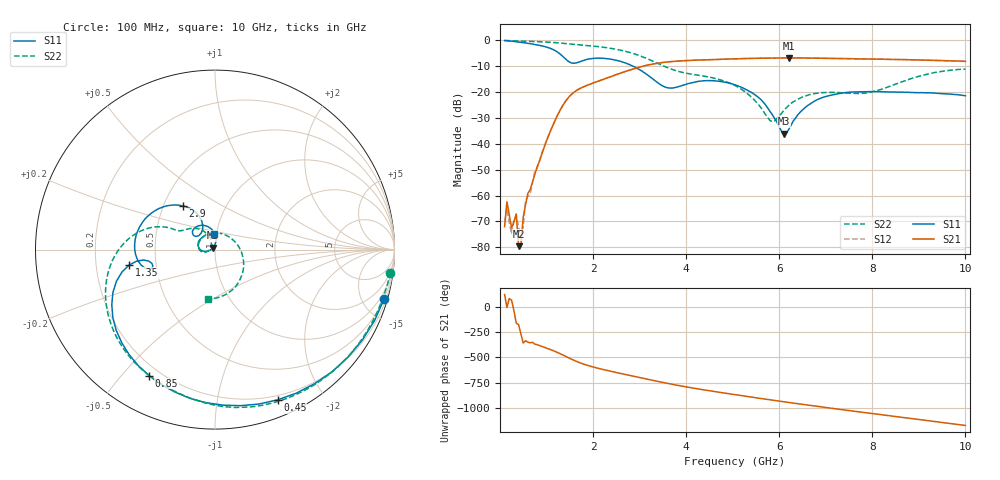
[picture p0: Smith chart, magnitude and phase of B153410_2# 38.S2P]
!  2-Port S-parameters saved by WinCal
! VAR MeasName=S-Parameters (CALIBRATED_DATA) read from VNA (N5245A)
! VAR MeasDate=2016-12-23 10:01:18
! VAR NAME=B153410_2# 38
! VAR FILENAME=B153410_2# 38.S2P
! VAR DATE=2016-12-23 10:01:18
! VAR PHYS_PORTS=1,2
# Hz S DB R 50
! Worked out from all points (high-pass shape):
!   199 points, 100 MHz to 10 GHz, reference 50 ohm
!   highest |S21| = -6.85 dB at 6.2 GHz (marker M1); lowest = -79.6 dB at 400 MHz (marker M2)
!   |S21| within 3 dB of the highest: 3.122 GHz to end of sweep
!   lowest |S11| = -36.1 dB at 6.1 GHz (marker M3), VSWR 1.03, Z = 49 + j1.14 ohm
!   |S11| at or under -10 dB: 2.852 GHz to end of sweep
!   |S22| runs from -31.5 to -0.1 dB; largest |S21 - S12| = 0.0033
!   S11 on the Smith chart (normalised r, x): 100 MHz: 0.46, -7.01; 450 MHz: 0.16, -1.49; 850 MHz: 0.16, -0.59; 1.35 GHz: 0.35, -0.08; 2.9 GHz: 0.63, +0.34; 10 GHz: 0.98, +0.17
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1e8  -0.16 -16.2  -72.01 124.3  -70.36 178.4  -0.13 -7.4
1.5e8  -0.24 -23.9  -62.42 -4.4  -64.98 -8.7  -0.17 -10.9
2.5e8  -0.42 -39.0  -72.53 68.3  -74.87 -42.4  -0.25 -17.7
3.5e8  -0.62 -53.5  -67.12 -160.2  -67.50 -9.8  -0.31 -24.3
4e8  -0.73 -60.5  -79.56 -174.6  -72.11 51.5  -0.33 -27.6
4.5e8  -0.85 -67.4  -79.07 93.5  -76.23 14.4  -0.36 -30.9
5e8  -0.97 -74.1  -68.38 2.5  -72.33 102.4  -0.39 -34.2
5.5e8  -1.10 -80.7  -63.50 25.7  -61.98 18.6  -0.42 -37.5
6e8  -1.23 -87.1  -59.14 11.3  -60.30 29.5  -0.45 -40.8
8.5e8  -2.02 -117.6  -46.75 -22.3  -46.40 -23.9  -0.63 -57.1
1.35e9  -6.27 -169.8  -25.25 -115.5  -25.25 -115.5  -1.21 -89.2
1.75e9  -8.11 -164.2  -18.41 160.8  -18.40 161.1  -1.89 -112.4
2.9e9  -10.42 126.1  -10.92 30.0  -10.92 29.9  -5.39 -179.8
3.4e9  -16.57 117.3  -8.88 -19.4  -8.87 -19.5  -9.06 158.9
4.15e9  -16.33 144.6  -7.78 -84.8  -7.78 -84.9  -13.24 151.2
5.05e9  -17.26 108.9  -7.23 -150.3  -7.24 -150.3  -17.52 124.5
5.8e9  -27.47 84.1  -6.93 158.9  -6.93 159.0  -31.03 143.8
6.1e9  -36.12 131.6  -6.86 139.1  -6.86 139.1  -27.09 -166.8
6.2e9  -34.63 169.1  -6.85 132.5  -6.87 132.5  -25.27 -164.9
6.7e9  -24.20 -171.2  -6.92 100.6  -6.94 100.5  -20.84 175.7
8.35e9  -20.03 143.3  -7.43 1.0  -7.42 0.9  -17.99 14.0
1e10  -21.49 92.4  -8.18 -96.1  -8.22 -95.9  -11.21 -97.7
